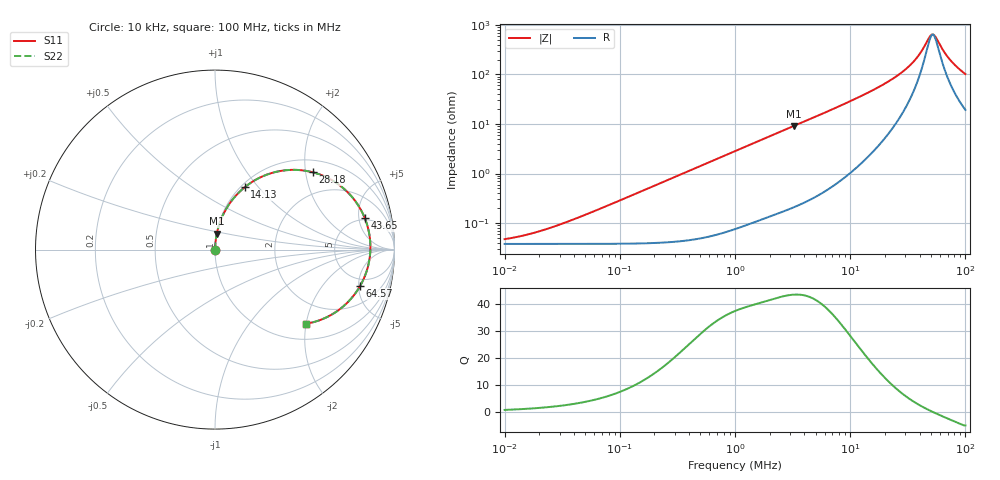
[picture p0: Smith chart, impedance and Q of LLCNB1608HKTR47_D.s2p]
! LLCNB1608HKTR47_D  S-PARAMETER MODEL  ( Standard Model )
! Model Generated by TAIYO YUDEN Corporation (http://www.ty-top.com)
! Version 1.0
! TAIYO YUDEN Control No. 200410
! Copyright(c) 2020 TAIYO YUDEN CO.,LTD. All Rights Reserved.
! Product Description (link to TY-COMPAS)
! https://ds.yuden.co.jp/TYCOMPAS/or/detail?pn=LLCNB1608HKTR47MD&u=M
! Products Name : Inductors
! Characteristics :
!  Inductance : 0.47 [uH] , SRF(min) : - [Hz] , DC Resistance(max) : 43 [mOhm]
!  Rated Current : Saturation  3.3 [A] (dL = 30 [%]), Temp Rise  2.7 [A] (dT = 40 [degC])
!  Case Size : 1.6 x 0.8 / 0.063 x 0.031 [mm/inch] , Thickness : 0.8 / 0.031 [mm/inch]
!  (Conditions: Temperature = 25 [degC] , DC Bias Current = 0 [A])
! External Node Assignments :
!  1  o---GGG---o  2
! GND o---------o GND
! Frequency Range : 10kHz  -  100MHz  [ 402 STEP ]
# MHz S RI R 50
! Freq[MHz].  S11 Real  S11 Imag  S21 Real  S21 Imag  S12 Real  S12 Imag  S22 Real  S22 Imag
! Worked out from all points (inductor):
!   401 points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, 10 kHz to 100 MHz, reference 50 ohm
!   read as one part in series: L = 452 nH near 40.74 kHz
!   highest Q = 43.4 at 3.236 MHz (marker M1), where L = 445 nH
!   self-resonance near 52.1 MHz
!   S11 on the Smith chart (normalised r, x): 10 kHz: 1.00, +0.00; 14.13 MHz: 1.04, +0.85; 28.18 MHz: 1.32, +2.20; 43.65 MHz: 4.72, +6.05; 64.57 MHz: 3.93, -5.22; 100 MHz: 1.39, -2.00
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0.01  0.00038 0.000283  0.9996 -0.000283  0.9996 -0.000283  0.00038 0.000283
0.019953  0.00038 0.000566  0.9996 -0.000566  0.9996 -0.000566  0.00038 0.000566
0.046774  0.000382 0.00133  0.9996 -0.00133  0.9996 -0.00133  0.000382 0.00133
0.218776  0.000439 0.0062  0.9996 -0.0062  0.9996 -0.0062  0.000439 0.0062
1  0.00155 0.0282  0.9985 -0.0282  0.9985 -0.0282  0.00155 0.0282
3.235937  0.0102 0.0894  0.9898 -0.0894  0.9898 -0.0894  0.0102 0.0894
4.677351  0.0199 0.1281  0.9801 -0.1281  0.9801 -0.1281  0.0199 0.1281
8.912509  0.0679 0.2359  0.9321 -0.2359  0.9321 -0.2359  0.0679 0.2359
14.12538  0.1649 0.3469  0.8351 -0.3469  0.8351 -0.3469  0.1649 0.3469
17.78279  0.2539 0.4031  0.7461 -0.4031  0.7461 -0.4031  0.2539 0.4031
21.87762  0.3669 0.4385  0.6331 -0.4385  0.6331 -0.4385  0.3669 0.4385
28.18383  0.5464 0.4303  0.4536 -0.4303  0.4536 -0.4303  0.5464 0.4303
36.30781  0.7363 0.3225  0.2637 -0.3225  0.2637 -0.3225  0.7363 0.3225
39.81072  0.7926 0.2548  0.2074 -0.2548  0.2074 -0.2548  0.7926 0.2548
43.65158  0.835 0.1744  0.165 -0.1744  0.165 -0.1744  0.835 0.1744
48.97788  0.8632 0.0623  0.1368 -0.0623  0.1368 -0.0623  0.8632 0.0623
52.48075  0.8654 -0.0074  0.1346 0.0074  0.1346 0.0074  0.8654 -0.0074
56.23413  0.8566 -0.0761  0.1434 0.0761  0.1434 0.0761  0.8566 -0.0761
64.56542  0.8086 -0.2025  0.1914 0.2025  0.1914 0.2025  0.8086 -0.2025
70.79458  0.7582 -0.2733  0.2418 0.2733  0.2418 0.2733  0.7582 -0.2733
79.43282  0.681 -0.3425  0.319 0.3425  0.319 0.3425  0.681 -0.3425
100  0.5079 -0.4127  0.4921 0.4127  0.4921 0.4127  0.5079 -0.4127
